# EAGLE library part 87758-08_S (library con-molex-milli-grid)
HEADER
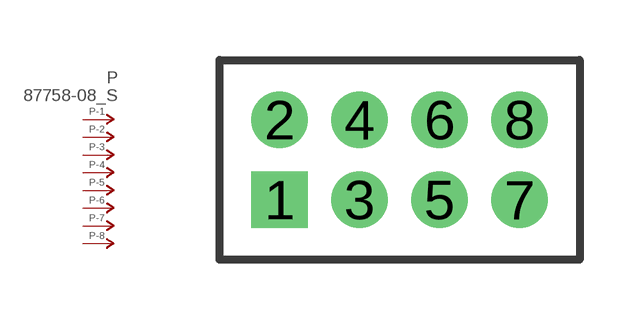
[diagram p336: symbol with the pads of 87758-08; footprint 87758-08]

Designator prefix P; gates -1=P-NV -2=P-N -3=P-N -4=P-N -5=P-N -6=P-N -7=P-N -8=P-N

## 87758-08_S  [87758-08]
1  -1:P  pas
2  -2:P  pas
3  -3:P  pas
4  -4:P  pas
5  -5:P  pas
6  -6:P  pas
7  -7:P  pas
8  -8:P  pas

## Footprint 87758-08 (pad centres in mm)
HEADER Dual Row, Vertical
drill 0.914 square: 1 -3,-1
drill 0.914: 2 -3,1; 3 -1,-1; 4 -1,1; 5 1,-1; 6 1,1; 7 3,-1; 8 3,1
